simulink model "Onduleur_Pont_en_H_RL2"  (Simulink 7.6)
settings: Solver=ode15s  StartTime=0.0  StopTime=30  RelTol=1e-3
InitFcn:
  | clc
  | clear all
StopFcn:
  | close all, clc
  | load Vitesse_Consigne_position.mat
  | plot(x(1,:),x(2,:),x(1,:),x(3,:),x(1,:),x(4,:))
  | xlabel('temps')
  | title('Consigne et vitesse de rotation')
  | grid
  | 
  | load Cde_Position.mat
  | figure
  | plot(y(1,:),y(2,:),y(1,:),y(3,:))
  | xlabel('temps')
  | title('Signal de commande PID')
  | grid
  | 
  | delete *.mat
undefined symbols (not defined in the file or in its folder): Ts
libraries: powerlib x15, fl_lib x11, nesl_utility x6, elec_lib x1, powerlib_extras x1

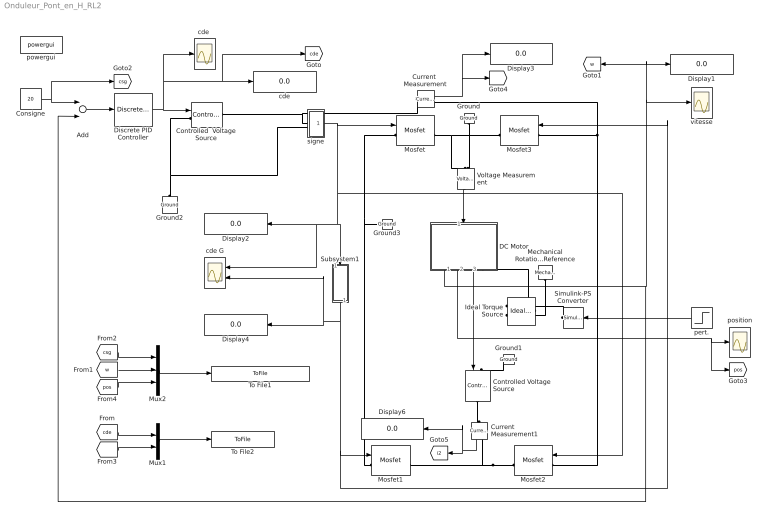
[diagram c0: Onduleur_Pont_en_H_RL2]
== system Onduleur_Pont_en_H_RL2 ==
  Add : Sum  Inputs=+-
  Consigne : Constant  Value=20
  Controlled  Voltage Source : powerlib/Electrical Sources/Controlled Voltage Source  DialogController=POWERSYS.PowerSysDialog  SystemSampleTime=-1  Initialize=on  Source_Type=AC  Amplitude=0  Phase=0  Frequency=0  Measurements=None
  Controlled Voltage Source : powerlib/Electrical Sources/Controlled Voltage Source  DialogController=POWERSYS.PowerSysDialog  SystemSampleTime=-1  Initialize=on  Source_Type=AC  Amplitude=0  Phase=0  Frequency=0  Measurements=None
  Current  Measurement : powerlib/Measurements/Current Measurement  DialogController=POWERSYS.PowerSysDialog  SystemSampleTime=-1  PhasorSimulation=off  OutputType=Complex  PSBequivalent=0
  Current  Measurement1 : powerlib/Measurements/Current Measurement  DialogController=POWERSYS.PowerSysDialog  SystemSampleTime=-1  PhasorSimulation=off  OutputType=Complex  PSBequivalent=0
  DC Motor : Subsystem
  Discrete PID Controller : powerlib_extras/Discrete  Control Blocks/Discrete PID Controller  DialogController=POWERSYS.PowerSysDialog  SystemSampleTime=-1  Kp=12  Ki=2  Kd=0  TcD=0  Par_Limits=[100 -100]  Init=0  Ts=5e-5
  Display{1..4,6} (5 alike) : Display
  Ground{,1..3} (4 alike) : powerlib/Elements/Ground  DialogController=POWERSYS.PowerSysDialog  PhysicalDomain=powersysdomain  SubClassName=unknown  LeftPortType=p1  RightPortType=p1  LConnTagsString=a
  Ideal Torque Source : fl_lib/Mechanical/Mechanical Sources/Ideal Torque Source  DialogController=NetworkEngine.DynNeDlgSource  SystemSampleTime=-1  w_Log=off  t_Log=off  LocalVarNames=|w|t  LocalVarDescs=|w|t  LocalVarLogging=[0 0]
  Mechanical Rotational Reference : fl_lib/Mechanical/Rotational Elements/Mechanical Rotational Reference  DialogController=NetworkEngine.DynNeDlgSource  SystemSampleTime=-1  t_Log=off  LocalVarNames=|t  LocalVarDescs=|t  LocalVarLogging=0
  Mosfet{,1..3} (4 alike) : powerlib/Power Electronics/Mosfet  DialogController=POWERSYS.PowerSysDialog  SystemSampleTime=-1  Ron=1e-6  Lon=0  Rd=0.001  Vfd=0  IC=0  Rs=1e8  Cs=inf  Measurements=on
  Mux1 : Mux  Inputs=2
  Mux2 : Mux  Inputs=3
  Simulink-PS Converter : nesl_utility/Simulink-PS Converter  DialogController=NetworkEngine.DynNeUtilDlgSource  SystemSampleTime=-1  PhysicalDomain=network_engine_domain  LeftPortType=input  RightPortType=output  SubClassName=ps_input  Unit=1  AffineConversion=off  InputFilterTimeConstant=.001  UdotUserProvided=0
  Subsystem1 : Subsystem
  To File1 : ToFile  Filename=Vitesse_Consigne_position  MatrixName=x
  To File2 : ToFile  Filename=Cde_Position  MatrixName=y
  Voltage Measurement : powerlib/Measurements/Voltage Measurement  DialogController=POWERSYS.PowerSysDialog  SystemSampleTime=-1  PhasorSimulation=off  OutputType=Complex  PSBequivalent=0
  cde : Display
  "cde " : Scope
  cde G : Scope  NumInputPorts=2
  pert. : Step  Time=25  Before=-0.001  After=0  SampleTime=0
  position : Scope
  powergui : powerlib/powergui  SystemSampleTime=-1  SimulationMode=Continuous  SampleTime=Ts  frequency=60  SPID=off  DisableSnubberDevices=off  DisableRonSwitches=off  DisableVfSwitches=off  SwTol=0  Interpol=off  frequencyindice=0  echomessages=off  HookPort=off  DisplayEquations=off  FunctionMessages=off  EnableUseOfTLC=off  x0status=blocks  RestoreLinks=warning  ResistiveCurrentMeasurement=off  Frange=[0:2:500]  Ylog=off  Xlog=on  ShowGrid=off  save=off  variable=ZData  ZoomFFT=on  StartTime=0.0  cycles=1  DisplayStyle=1  fundamental=60  FreqAxis=off  MaxFrequency=1000  frequencyindicesteady=1  RmsSteady=1  display=off  Ts=0  methode=off
  signe : Subsystem
  vitesse : Scope
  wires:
  Subsystem1/1(1-2u) -> Mosfet1/1, Mosfet3/1, Display4/1, cde G/2
  Voltage Measurement/1 -> DC Motor/1(U+)
  DC Motor/2(alpha) -> position/1, [pos]
  Add/1 -> Discrete PID Controller/1
  Consigne/1 -> [csg], Add/1
  signe/1(sgn) -> Mosfet2/1, Subsystem1/1(u), Display2/1, cde G/1, Mosfet/1
  DC Motor/1(w) -> Add/2, vitesse/1, [w], Display1/1
  Discrete PID Controller/1 -> Controlled  Voltage Source/1, "cde "/1, cde/1, [cde]
  pert./1 -> Simulink-PS Converter/1
  [w] -> Mux2/2
  Mux2/1 -> To File1/1
  [csg] -> Mux2/1
  [pos] -> Mux2/3
  Current  Measurement/1 -> [i], Display3/1
  [cde] -> Mux1/1
  [i] -> Mux1/2
  Mux1/1 -> To File2/1
  DC Motor/3(U-) -> Controlled Voltage Source/1
  Current  Measurement1/1 -> [i2], Display6/1
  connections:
  Mosfet2/RConn1 -- Mosfet1/RConn1 -- Current  Measurement1/RConn1
  Mosfet/RConn1 -- Mosfet3/RConn1 -- Voltage Measurement/LConn1
  Ground/LConn1 -- Voltage Measurement/LConn2
  Ground1/LConn1 -- Controlled Voltage Source/LConn1
  Mosfet1/LConn1 -- Mosfet/LConn1 -- Ground3/LConn1
  Ideal Torque Source/LConn1 -- DC Motor/RConn1
  Simulink-PS Converter/RConn1 -- Ideal Torque Source/RConn1
  Mosfet2/LConn1 -- Mosfet3/LConn1 -- Current  Measurement/RConn1
  Mechanical Rotational Reference/LConn1 -- Ideal Torque Source/RConn2
  signe/LConn1 -- Controlled  Voltage Source/RConn1 -- Current  Measurement/LConn1
  Controlled Voltage Source/RConn1 -- Current  Measurement1/LConn1
  Ground2/LConn1 -- Controlled  Voltage Source/LConn1 -- signe/LConn2

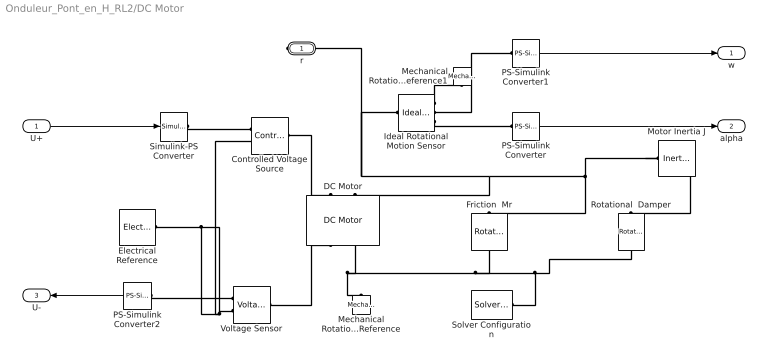
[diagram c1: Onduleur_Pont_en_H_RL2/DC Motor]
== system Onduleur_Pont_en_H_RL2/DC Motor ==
  U+ : Inport
  Controlled Voltage Source : fl_lib/Electrical/Electrical Sources/Controlled Voltage Source  DialogController=NetworkEngine.DynNeDlgSource  SystemSampleTime=-1  i_Log=off  v_Log=off  LocalVarNames=|i|v  LocalVarDescs=|i|v  LocalVarLogging=[0 0]
  DC Motor : elec_lib/Actuators & Drivers/Rotational Actuators/DC Motor  DialogController=NetworkEngine.DynNeDlgSource  SystemSampleTime=-1  parameterization=1  Ra=3.9 Ohm  La=1.2e-3 H  emf_or_torque=2  Kv=7.2e-5 V/rpm  Ki=10e-3 N*m/A  T_stall=2.4e-4 N*m  w_max=1.91e+4 rpm  w_rated=1.5e+4 rpm  P_rated=0.08 W  V_rated=1.5 V  J=0.01 g*cm^2  lam=1e-8 N*m/(rad/s)  speed0=0 rpm  current_Log=off  voltage_Log=off  power_Log=off  i2r_Log=off  torque_Log=off  speed_Log=off  LocalVarNames=|current|voltage|power|i2r|torque|speed  LocalVarDescs=|Current (A)|Voltage (V)|Power (W)|Electrical losses (W)|Torque (Nm)|Angular speed (rad/s)  LocalVarLogging=[0 0 0 0 0 0]
  Electrical Reference : fl_lib/Electrical/Electrical Elements/Electrical Reference  DialogController=NetworkEngine.DynNeDlgSource  SystemSampleTime=-1  i_Log=off  LocalVarNames=|i  LocalVarDescs=|i  LocalVarLogging=0
  Friction  Mr : fl_lib/Mechanical/Rotational Elements/Rotational Friction  DialogController=NetworkEngine.DynNeDlgSource  SystemSampleTime=-1  brkwy_trq=0.01e-3 N*m  Col_trq=0.01e-3 N*m  visc_coef=0.001e-3 N*m/(rad/s)  trans_coef=10 s/rad  vel_thr=0.1 rad/s  t_Log=off  w_Log=off  LocalVarNames=|friction_torque|rel_velocity|power  LocalVarDescs=|Friction torque (N*m)|Relative velocity (rad/s)|Power (W)  LocalVarLogging=[0 0 0]
  Ideal Rotational Motion Sensor : fl_lib/Mechanical/Mechanical Sensors/Ideal Rotational Motion Sensor  DialogController=NetworkEngine.DynNeDlgSource  SystemSampleTime=-1  offset=0 rad  w_Log=off  t_Log=off  phi_Log=off  LocalVarNames=|w|t|phi  LocalVarDescs=|w|t|phi  LocalVarLogging=[0 0 0]
  Mechanical Rotational Reference : fl_lib/Mechanical/Rotational Elements/Mechanical Rotational Reference  DialogController=NetworkEngine.DynNeDlgSource  SystemSampleTime=-1  t_Log=off  LocalVarNames=|t  LocalVarDescs=|t  LocalVarLogging=0
  Mechanical Rotational Reference1 : fl_lib/Mechanical/Rotational Elements/Mechanical Rotational Reference  DialogController=NetworkEngine.DynNeDlgSource  SystemSampleTime=-1  t_Log=off  LocalVarNames=|t  LocalVarDescs=|t  LocalVarLogging=0
  Motor Inertia J : fl_lib/Mechanical/Rotational Elements/Inertia  DialogController=NetworkEngine.DynNeDlgSource  SystemSampleTime=-1  inertia=0.001 g*cm^2  initial_velocity=0 rad/s  t_Log=off  LocalVarNames=|torque|velocity  LocalVarDescs=|Inertia torque (N*m)|Inertia absolute velocity (rad/s)  LocalVarLogging=[0 0]
  PS-Simulink Converter : nesl_utility/PS-Simulink Converter  DialogController=NetworkEngine.DynNeUtilDlgSource  SystemSampleTime=-1  PhysicalDomain=network_engine_domain  LeftPortType=input  RightPortType=output  SubClassName=ps_output  Unit=1  AffineConversion=off
  PS-Simulink Converter1 : nesl_utility/PS-Simulink Converter  DialogController=NetworkEngine.DynNeUtilDlgSource  SystemSampleTime=-1  PhysicalDomain=network_engine_domain  LeftPortType=input  RightPortType=output  SubClassName=ps_output  Unit=1  AffineConversion=off
  PS-Simulink Converter2 : nesl_utility/PS-Simulink Converter  DialogController=NetworkEngine.DynNeUtilDlgSource  SystemSampleTime=-1  PhysicalDomain=network_engine_domain  LeftPortType=input  RightPortType=output  SubClassName=ps_output  Unit=1  AffineConversion=on
  Rotational  Damper : fl_lib/Mechanical/Rotational Elements/Rotational Damper  DialogController=NetworkEngine.DynNeDlgSource  SystemSampleTime=-1  D=0.001 N*m/(rad/s)  t_Log=off  w_Log=off  LocalVarNames=|t|w  LocalVarDescs=|t|w  LocalVarLogging=[0 0]
  Simulink-PS Converter : nesl_utility/Simulink-PS Converter  DialogController=NetworkEngine.DynNeUtilDlgSource  SystemSampleTime=-1  PhysicalDomain=network_engine_domain  LeftPortType=input  RightPortType=output  SubClassName=ps_input  Unit=1  AffineConversion=off  InputFilterTimeConstant=.001  UdotUserProvided=0
  Solver Configuration : nesl_utility/Solver Configuration  DialogController=NetworkEngine.DynNeUtilDlgSource  SystemSampleTime=-1  PhysicalDomain=network_engine_domain  LeftPortType=input  RightPortType=generic  SubClassName=solver  Accelerate=off  Profile=off  ResidualTolerance=1e-9  MaxNonlinIter=3  MaxModeIter=2  DoFixedCost=off  UseLocalSampling=off  DoDC=off  LinearAlgebra=Sparse  LocalSolverSampleTime=.001  LocalSolverChoice=NE_BACKWARD_EULER_ADVANCER  UseLocalSolver=off
  Voltage Sensor : fl_lib/Electrical/Electrical Sensors/Voltage Sensor  DialogController=NetworkEngine.DynNeDlgSource  SystemSampleTime=-1  i1_Log=off  v1_Log=off  LocalVarNames=|i1|v1  LocalVarDescs=|i1|v1  LocalVarLogging=[0 0]
  r : PMIOPort  Port=1  Side=Right
  w : Outport
  alpha : Outport  Port=2
  U- : Outport  Port=3
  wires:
  U+/1 -> Simulink-PS Converter/1
  PS-Simulink Converter/1 -> alpha/1
  PS-Simulink Converter1/1 -> w/1
  PS-Simulink Converter2/1 -> U-/1
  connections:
  Ideal Rotational Motion Sensor/RConn3 -- PS-Simulink Converter/LConn1
  Ideal Rotational Motion Sensor/RConn2 -- PS-Simulink Converter1/LConn1
  Ideal Rotational Motion Sensor/RConn1 -- Mechanical Rotational Reference1/LConn1
  Solver Configuration/RConn1 -- Rotational  Damper/RConn1 -- Friction  Mr/RConn1 -- DC Motor/RConn2 -- Mechanical Rotational Reference/LConn1
  Motor Inertia J/LConn1 -- Rotational  Damper/LConn1 -- Friction  Mr/LConn1 -- DC Motor/LConn2 -- r/RConn1 -- Ideal Rotational Motion Sensor/LConn1
  PS-Simulink Converter2/LConn1 -- Voltage Sensor/RConn1
  Voltage Sensor/LConn1 -- DC Motor/RConn1
  Voltage Sensor/RConn2 -- Controlled Voltage Source/RConn2 -- Electrical Reference/LConn1
  Simulink-PS Converter/RConn1 -- Controlled Voltage Source/RConn1
  Controlled Voltage Source/LConn1 -- DC Motor/LConn1

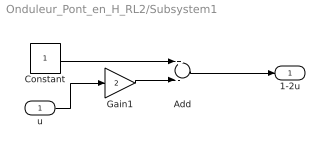
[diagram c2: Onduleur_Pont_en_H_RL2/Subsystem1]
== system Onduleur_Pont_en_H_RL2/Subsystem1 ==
  u : Inport
  Add : Sum  Inputs=+-
  Constant : Constant
  Gain1 : Gain  Gain=2
  1-2u : Outport
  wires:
  u/1 -> Gain1/1
  Add/1 -> 1-2u/1
  Constant/1 -> Add/1
  Gain1/1 -> Add/2

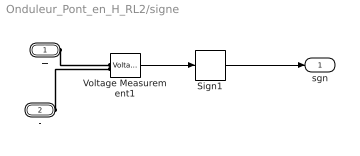
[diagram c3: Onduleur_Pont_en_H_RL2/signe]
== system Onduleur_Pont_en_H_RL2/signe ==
  Sign1 : Signum
  Voltage Measurement1 : powerlib/Measurements/Voltage Measurement  DialogController=POWERSYS.PowerSysDialog  SystemSampleTime=-1  PhasorSimulation=off  OutputType=Complex  PSBequivalent=0
  + : PMIOPort  Port=1  Side=Left
  - : PMIOPort  Port=2  Side=Left
  sgn : Outport
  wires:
  Voltage Measurement1/1 -> Sign1/1
  Sign1/1 -> sgn/1
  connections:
  +/RConn1 -- Voltage Measurement1/LConn1
  -/RConn1 -- Voltage Measurement1/LConn2
